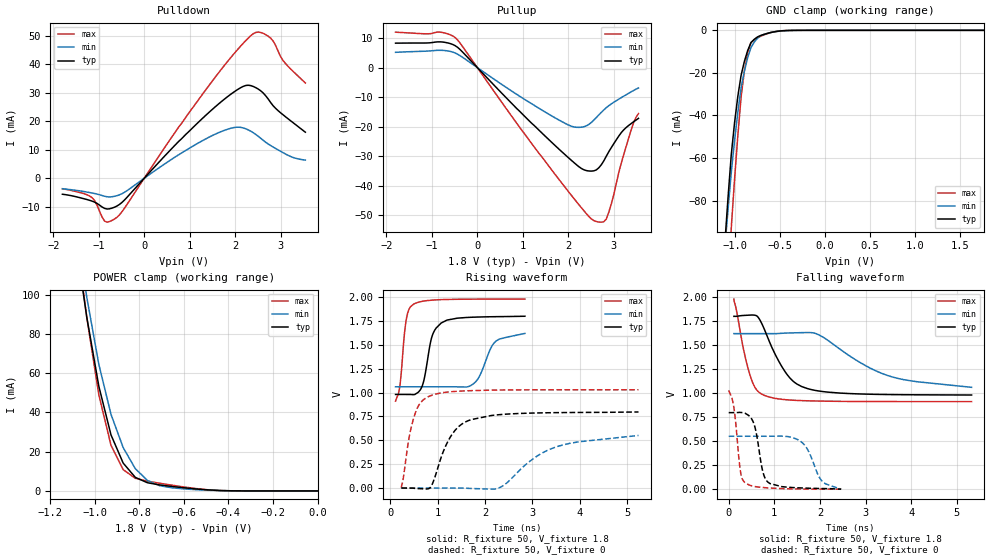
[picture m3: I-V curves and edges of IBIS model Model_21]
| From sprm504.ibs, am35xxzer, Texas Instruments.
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| Model based on original model for BC1833DV65ATPBFHP18LL_7LM_X50
|   Sub model LM_X50_PD_PU_OFF_1P8
[model]   Model_21
|[Description]  1.8V-I/O-PI-X
|[Input Load]   PI
|[Output Drive]
|Voltage   1.8V
|Mode   I/O
Model_type   I/O
Polarity   Non-Inverting
Enable   Active-Low
Vinl =  0.63V
Vinh =  1.17V
Cref =  15pF
Rref =  100.0000M
Vref =  0V
Vmeas =  0.9
C_comp   1.827006p   1.710031p   1.865433p
[Model Spec]
Vinl   0.63V   0.567V   0.693V
Vinh   1.17V   1.053V   1.287V
[Temperature Range]   25   125   -40
[Voltage Range]   1.8   1.62   1.98
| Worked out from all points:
|   slope of the pulldown table from 0 to 0.27 V, typ, clamps not added: 57.3 ohm
|   slope of the pullup table from 0 to 0.27 V, typ, clamps not added: 61.7 ohm
|   GND clamp passes 1 mA (typ) near -0.59 V on its own axis
|   POWER clamp passes 1 mA (typ) near -0.55 V on its own axis
|   rising waveform, R_fixture 50, V_fixture 1.8: 20-80 % time 203ps typ, 290ps min, 123ps max; typ from 0.981 V to 1.8 V
|   rising waveform, R_fixture 50, V_fixture 0: 20-80 % time 459ps typ, 984ps min, 254ps max; typ from 0 V to 0.797 V
|   falling waveform, R_fixture 50, V_fixture 1.8: 20-80 % time 561ps typ, 1.26ns min, 304ps max; typ from 1.8 V to 0.981 V
|   falling waveform, R_fixture 50, V_fixture 0: 20-80 % time 182ps typ, 311ps min, 130ps max; typ from 0.797 V to 0 V
[POWER_clamp]
-1.8V     828.5mA    859.7mA    895.1mA
-1.055V   103mA      112.7mA    104.7mA
-1.036V   88.74mA    98.85mA    88.62mA
-981.8mV  53.26mA    64.41mA    48.86mA
-927.3mV  28.53mA    39.01mA    23.24mA
-872.7mV  14.2mA     22.1mA     10.86mA
-818.2mV  6.917mA    11.35mA    6.446mA
-763.6mV  4.168mA    5.31mA     4.979mA
-709.1mV  3.063mA    2.677mA    3.924mA
-545.5mV  1.001mA    625.3uA    1.212mA
-381.8mV  59.21uA    52.93uA    42.45uA
0V        17.79nA    60.71nA    29.21nA
[Pulldown]
-1.8V     -5.591mA   -3.681mA   -3.662mA
-1.145V   -8.02mA    -5.175mA   -6.828mA
-872.7mV  -10.55mA   -6.29mA    -14.99mA
-600mV    -9.724mA   -6.096mA   -13.67mA
709.1mV   12.12mA    7.769mA    16.82mA
1.636V    26.06mA    15.99mA    36.98mA
1.964V    30.14mA    17.75mA    43.45mA
2.182V    32.24mA    17.64mA    47.39mA
2.455V    31.77mA    15.36mA    51.13mA
2.782V    26.55mA    11.48mA    49.14mA
3.055V    22.26mA    8.979mA    41.29mA
3.545V    16.16mA    6.369mA    33.41mA
[Pullup]
-1.8V     8.287mA    5.179mA    12.01mA
-818.2mV  8.728mA    5.865mA    12.02mA
-490.9mV  7.457mA    4.972mA    10.2mA
2.018V    -30.72mA   -19.53mA   -42.27mA
2.345V    -34.62mA   -20.02mA   -48.51mA
2.618V    -34.65mA   -16.89mA   -52.16mA
2.836V    -30.05mA   -13.59mA   -51.31mA
2.945V    -27.15mA   -12.31mA   -46.28mA
3.164V    -22.09mA   -10.2mA    -32.55mA
3.327V    -19.63mA   -8.709mA   -23.98mA
3.436V    -18.37mA   -7.753mA   -18.75mA
3.545V    -17.2mA    -6.896mA   -15.57mA
[GND_clamp]
-1.8V     -653mA     -527.8mA   -1.091A
-1.109V   -100.9mA   -102.8mA   -157.8mA
-1.073V   -78.75mA   -84.4mA    -123.2mA
-1.036V   -58.39mA   -66.85mA   -92.81mA
-1V       -43.41mA   -51.82mA   -69.99mA
-927.3mV  -21.09mA   -26.93mA   -31.24mA
-890.9mV  -14.57mA   -19.13mA   -18.96mA
-854.5mV  -9.47mA    -12.85mA   -10.46mA
-818.2mV  -5.796mA   -8.117mA   -5.718mA
-745.5mV  -3.105mA   -3.688mA   -3.474mA
-381.8mV  -52.95uA   -71.88uA   -53.31uA
1.764V    17.39nA    304.1nA    24.84nA
[Ramp]
dV/dt_f 0.49989371/0.56498023n 0.34245875/1.2706881n 0.64840596/0.30536819n
dV/dt_r 0.48412499/0.4590658n 0.33767456/0.98693342n 0.62234659/0.25437822n
R_load = 50
[Rising Waveform]
R_fixture = 50
V_fixture = 1.8
V_fixture_min = 1.62
V_fixture_max = 1.98
109.8ps   980.7mV    1.061V     911.9mV
201.1ps   980.7mV    1.061V     1.072V
342.1ps   980.5mV    1.061V     1.78V
495.7ps   978.5mV    1.061V     1.928V
671.2ps   1.067V     1.061V     1.956V
874.7ps   1.58V      1.061V     1.968V
1.072ns   1.728V     1.061V     1.974V
1.708ns   1.789V     1.077V     1.979V
2.202ns   1.795V     1.526V     1.98V
2.842ns   1.8V       1.62V      1.98V
[Rising Waveform]
R_fixture = 50
V_fixture = 0
V_fixture_min = 0
V_fixture_max = 0
233.5ps   9.932nV    86.12nV    12nV
386.7ps   -266.9uV   -773.9nV   502.5mV
479.3ps   -817.6uV   -711.8nV   710.5mV
624ps     -6.357mV   484.1nV    885.2mV
837.6ps   3.046mV    740.7nV    965mV
1.26ns    529mV      -22.58uV   1.008V
1.698ns   716.1mV    -4.127mV   1.02V
2.306ns   768.9mV    4.379mV    1.027V
3.569ns   790.4mV    441.7mV    1.029V
5.241ns   797.1mV    551.2mV    1.03V
[Falling Waveform]
R_fixture = 50
V_fixture = 1.8
V_fixture_min = 1.62
V_fixture_max = 1.98
114.8ps   1.8V       1.62V      1.98V
332.5ps   1.809V     1.62V      1.441V
473.5ps   1.813V     1.62V      1.178V
634ps     1.797V     1.62V      1.023V
786.9ps   1.66V      1.62V      975.9mV
1.265ns   1.204V     1.626V     931.2mV
1.718ns   1.049V     1.631V     920.5mV
2.007ns   1.02V      1.599V     917.5mV
3.475ns   985.7mV    1.185V     912.3mV
5.322ns   980.7mV    1.061V     911.9mV
[Falling Waveform]
R_fixture = 50
V_fixture = 0
V_fixture_min = 0
V_fixture_max = 0
0s        797.1mV    551.2mV    1.03V
114.5ps   797.4mV    551.1mV    848.1mV
266.2ps   798.9mV    551.2mV    162mV
355.5ps   790.9mV    551.2mV    68.61mV
561.8ps   668.2mV    551.2mV    28.74mV
739.6ps   199.5mV    551.1mV    17.41mV
853.1ps   76.18mV    551mV      13.38mV
1.574ns   13.05mV    498.5mV    1.831mV
2.03ns    6.682mV    92.31mV    508.1uV
2.464ns   9.932nV    86.12nV    12nV
